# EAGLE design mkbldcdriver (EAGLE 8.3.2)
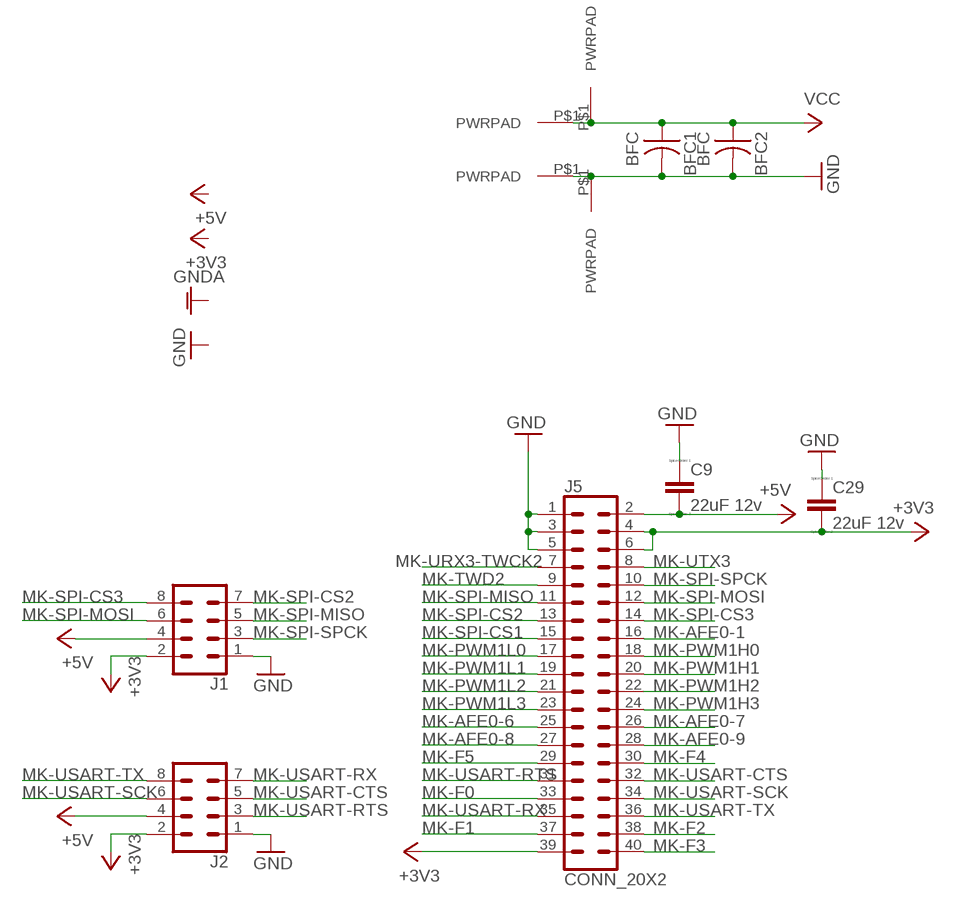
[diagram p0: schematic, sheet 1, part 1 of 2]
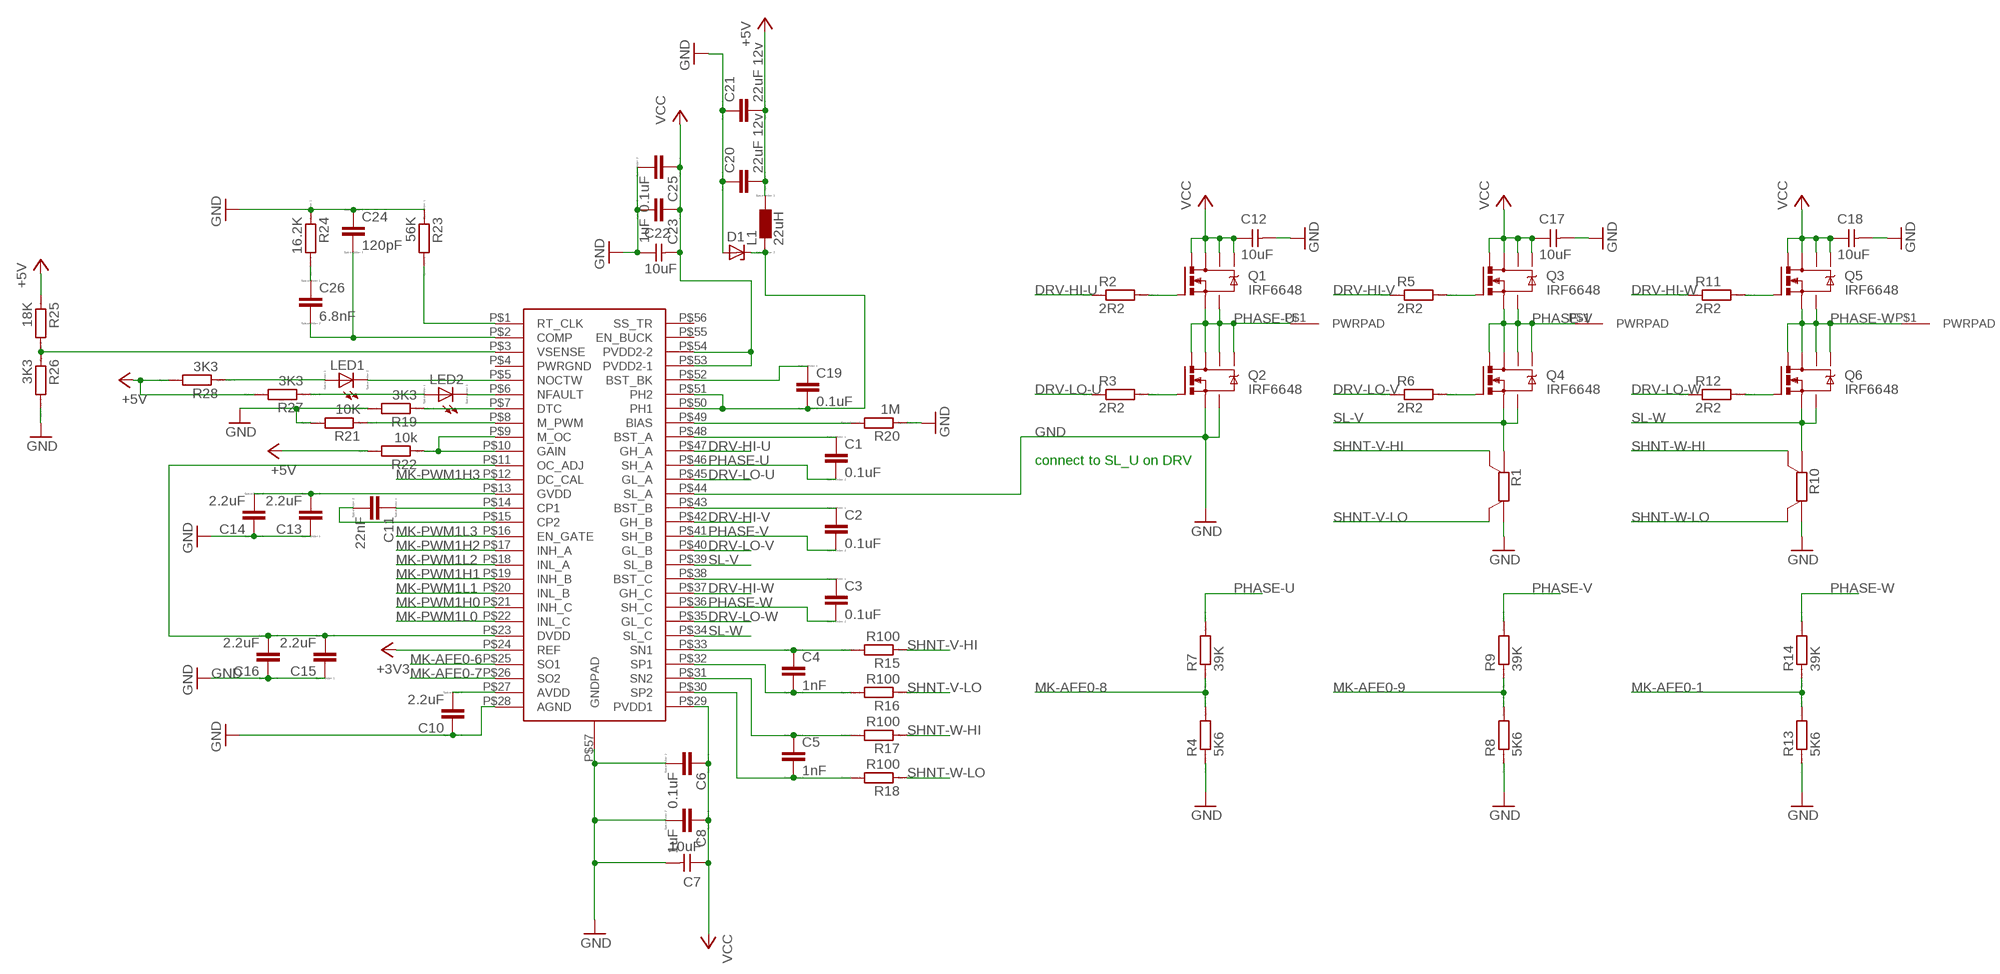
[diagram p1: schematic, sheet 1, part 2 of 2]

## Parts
BFC1  BFC  [BFC]
BFC2  BFC  [BFC]
C1  0.1uF  C  [C0805]
C2  0.1uF  C  [C0805]
C3  0.1uF  C  [C0805]
C4  1nF  C  [C0805]
C5  1nF  C  [C0805]
C6  0.1uF  C  [C0805]
C7  10uF  CAP-UNPOLARIZED2220  [C2220]
C8  1uF  C  [C0805]
C9  22uF 12v  C  [C0805]
C10  2.2uF  C  [C0805]
C11  22nF  C  [C0805]
C12  10uF  CAP-UNPOLARIZED2220  [C2220]
C13  2.2uF  C  [C0805]
C14  2.2uF  C  [C0805]
C15  2.2uF  C  [C0805]
C16  2.2uF  C  [C0805]
C17  10uF  CAP-UNPOLARIZED2220  [C2220]
C18  10uF  CAP-UNPOLARIZED2220  [C2220]
C19  0.1uF  C  [C0805]
C20  22uF 12v  C  [C0805]
C21  22uF 12v  C  [C0805]
C22  10uF  CAP-UNPOLARIZED2220  [C2220]
C23  1uF  C  [C0805]
C24  120pF  C  [C0805]
C25  0.1uF  C  [C0805]
C26  6.8nF  C  [C0805]
C29  22uF 12v  C  [C0805]
D1  ZENER_DIODESOD123  [SOD123]
J1  CONN_04X2SHROUDED  [2X4-SHROUDED]
J2  CONN_04X2SHROUDED  [2X4-SHROUDED]
J3  PWRPAD2-5MM  [PWRPAD_2-5MM]
J4  PWRPAD2-5MM  [PWRPAD_2-5MM]
J5  CONN_20X2  [2X20]
J6  PWRPAD2-5MM  [PWRPAD_2-5MM]
J7  PWRPAD4MM  [PWRPAD_4MM]
J8  PWRPAD4MM  [PWRPAD_4MM]
J9  PWRPAD4MM  [PWRPAD_4MM]
J10  PWRPAD4MM  [PWRPAD_4MM]
L1  22uH  L  [L1812]
LED1  LED_E  [LED_1206]
LED2  LED_E  [LED_1206]
Q1  IRF6648  [DIRECTFET]
Q2  IRF6648  [DIRECTFET]
Q3  IRF6648  [DIRECTFET]
Q4  IRF6648  [DIRECTFET]
Q5  IRF6648  [DIRECTFET]
Q6  IRF6648  [DIRECTFET]
R1  WSL2726  [WSL2726]
R2  2R2  R  [R0805]
R3  2R2  R  [R0805]
R4  5K6  R  [R0805]
R5  2R2  R  [R0805]
R6  2R2  R  [R0805]
R7  39K  R  [R0805]
R8  5K6  R  [R0805]
R9  39K  R  [R0805]
R10  WSL2726  [WSL2726]
R11  2R2  R  [R0805]
R12  2R2  R  [R0805]
R13  5K6  R  [R0805]
R14  39K  R  [R0805]
R15  R100  R  [R0805]
R16  R100  R  [R0805]
R17  R100  R  [R0805]
R18  R100  R  [R0805]
R19  3K3  R  [R0805]
R20  1M  R  [R0805]
R21  10K  R  [R0805]
R22  10k  R  [R0805]
R23  56K  R  [R0805]
R24  16.2K  R  [R0805]
R25  18K  R  [R0805]
R26  3K3  R  [R0805]
R27  3K3  R  [R0805]
R28  3K3  R  [R0805]
U$1  DRV8302  [HTSSOP-56]

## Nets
+3V3: C29.2 J1.2 J2.2 J5.4 J5.6 J5.39 U$1.P$24(REF)
+5V: C9.2 C20.2 C21.2 J1.4 J2.4 J5.2 L1.1 R22.2 R25.1 R27.2 R28.2
DRV-HI-U: R2.1 U$1.P$47(GH_A)
DRV-HI-V: R5.1 U$1.P$42(GH_B)
DRV-HI-W: R11.1 U$1.P$37(GH_C)
DRV-LO-U: R3.1 U$1.P$45(GL_A)
DRV-LO-V: R6.1 U$1.P$40(GL_B)
DRV-LO-W: R12.1 U$1.P$35(GL_C)
GND: BFC1.P$2 BFC2.P$2 C6.2 C7.2 C8.2 C9.1 C10.1 C12.2 C13.1 C14.1 C15.1 C16.1 C17.2 C18.2 C20.1 C21.1 C22.1 C23.2 C24.1 C25.2 C29.1 D1.ANODE J1.1 J2.1 J5.1 J5.3 J5.5 J8.P$1(PWRPAD) J10.P$1(PWRPAD) Q2.S@1(S) Q2.S@2(S) R1.A R4.1 R8.1 R10.A R13.1 R19.2 R20.1 R21.2 R23.1 R24.1 R26.2 U$1.P$28(AGND) U$1.P$44(SL_A) U$1.P$57(GNDPAD)
MK-AFE0-1: J5.16 R13.2 R14.1
MK-AFE0-6: J5.25 U$1.P$25(SO1)
MK-AFE0-7: J5.26 U$1.P$26(SO2)
MK-AFE0-8: J5.27 R4.2 R7.1
MK-AFE0-9: J5.28 R8.2 R9.1
MK-F0: J5.33
MK-F1: J5.37
MK-F2: J5.38
MK-F3: J5.40
MK-F4: J5.30
MK-F5: J5.29
MK-PWM1H0: J5.18 U$1.P$21(INH_C)
MK-PWM1H1: J5.20 U$1.P$19(INH_B)
MK-PWM1H2: J5.22 U$1.P$17(INH_A)
MK-PWM1H3: J5.24 U$1.P$12(DC_CAL)
MK-PWM1L0: J5.17 U$1.P$22(INL_C)
MK-PWM1L1: J5.19 U$1.P$20(INL_B)
MK-PWM1L2: J5.21 U$1.P$18(INL_A)
MK-PWM1L3: J5.23 U$1.P$16(EN_GATE)
MK-SPI-CS1: J5.15
MK-SPI-CS2: J1.7 J5.13
MK-SPI-CS3: J1.8 J5.14
MK-SPI-MISO: J1.5 J5.11
MK-SPI-MOSI: J1.6 J5.12
MK-SPI-SPCK: J1.3 J5.10
MK-TWD2: J5.9
MK-URX3-TWCK2: J5.7
MK-USART-CTS: J2.5 J5.32
MK-USART-RTS: J2.3 J5.31
MK-USART-RX: J2.7 J5.35
MK-USART-SCK: J2.6 J5.34
MK-USART-TX: J2.8 J5.36
MK-UTX3: J5.8
N$1: Q4.G R6.2
N$2: Q2.G R3.2
N$3: Q1.G R2.2
N$4: Q3.G R5.2
N$5: Q6.G R12.2
N$6: Q5.G R11.2
N$7: C3.1 U$1.P$38(BST_C)
N$8: C2.1 U$1.P$43(BST_B)
N$9: C1.1 U$1.P$48(BST_A)
N$11: C10.2 U$1.P$27(AVDD)
N$12: C11.1 U$1.P$14(CP1)
N$13: C4.1 R15.2 U$1.P$33(SN1)
N$14: C4.2 R16.2 U$1.P$32(SP1)
N$15: C5.1 R17.2 U$1.P$31(SN2)
N$16: C5.2 R18.2 U$1.P$30(SP2)
N$17: C11.2 U$1.P$15(CP2)
N$18: C13.2 C14.2 U$1.P$13(GVDD)
N$20: C15.2 C16.2 U$1.P$11(OC_ADJ) U$1.P$23(DVDD)
N$21: R19.1 U$1.P$7(DTC)
N$23: C19.1 U$1.P$52(BST_BK)
N$24: R20.2 U$1.P$49(BIAS)
N$25: R21.1 U$1.P$8(M_PWM)
N$26: R22.1 U$1.P$9(M_OC) U$1.P$10(GAIN)
N$27: C19.2 D1.CATHODE L1.2 U$1.P$50(PH1) U$1.P$51(PH2)
N$30: R23.2 U$1.P$1(RT_CLK)
N$31: C24.2 C26.2 U$1.P$2(COMP)
N$32: C26.1 R24.2
N$33: R25.2 R26.1 U$1.P$3(VSENSE)
N$35: LED1.C U$1.P$5(NOCTW)
N$36: LED2.C U$1.P$6(NFAULT)
N$37: LED2.A R27.1
N$38: LED1.A R28.1
PHASE-U: C1.2 J3.P$1(PWRPAD) Q1.S@1(S) Q1.S@2(S) Q2.D@1(D) Q2.D@2(D) Q2.D@3(D) Q2.D@4(D) R7.2 U$1.P$46(SH_A)
PHASE-V: C2.2 J4.P$1(PWRPAD) Q3.S@1(S) Q3.S@2(S) Q4.D@1(D) Q4.D@2(D) Q4.D@3(D) Q4.D@4(D) R9.2 U$1.P$41(SH_B)
PHASE-W: C3.2 J6.P$1(PWRPAD) Q5.S@1(S) Q5.S@2(S) Q6.D@1(D) Q6.D@2(D) Q6.D@3(D) Q6.D@4(D) R14.2 U$1.P$36(SH_C)
SHNT-V-HI: R1.SB R15.1
SHNT-V-LO: R1.SA R16.1
SHNT-W-HI: R10.SB R17.1
SHNT-W-LO: R10.SA R18.1
SL-V: Q4.S@1(S) Q4.S@2(S) R1.B U$1.P$39(SL_B)
SL-W: Q6.S@1(S) Q6.S@2(S) R10.B U$1.P$34(SL_C)
VCC: BFC1.P$1 BFC2.P$1 C6.1 C7.1 C8.1 C12.1 C17.1 C18.1 C22.2 C23.1 C25.1 J7.P$1(PWRPAD) J9.P$1(PWRPAD) Q1.D@1(D) Q1.D@2(D) Q1.D@3(D) Q1.D@4(D) Q3.D@1(D) Q3.D@2(D) Q3.D@3(D) Q3.D@4(D) Q5.D@1(D) Q5.D@2(D) Q5.D@3(D) Q5.D@4(D) U$1.P$29(PVDD1) U$1.P$53(PVDD2-1) U$1.P$54(PVDD2-2)
Unconnected: U$1.P$4(PWRGND) U$1.P$55(EN_BUCK) U$1.P$56(SS_TR)

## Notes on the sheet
- connect to SL_U on DRV

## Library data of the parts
BFC1 BFC2 = fab:BFC
C1-C6 C8-C11 C13-C16 C19-C21 C23-C26 C29 = eagle-ltspice:C: CAPACITOR, European symbol; SPICEMODEL: NONE; SPICEPREFIX: C
C7 C12 C17 C18 C22 = fab:CAP-UNPOLARIZED
D1 = fab:ZENER_DIODE: zener diode
J1 J2 = fab:CONN_04X2: Multi connection point. Often used as Generic Header-pin footprint for 0.1 inch spaced/style header connections On any of the 0.1 inch spaced packages, you can populate with these: Break Away Headers - Straight (PRT-00116) Break Away Male Headers - Right Angle (PRT-00553) Female Headers (PRT-00115)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
J3 J4 J6-J10 = fab:PWRPAD
J5 = SparkFun-Connectors:CONN_20X2: Multi connection point. Often used as Generic Header-pin footprint for 0.1 inch spaced/style header connections On any of the 0.1 inch spaced packages, you can populate with these: Break Away Headers - Straight (PRT-00116) Break Away Male Headers - Right Angle (PRT-00553) Female Headers (PRT-00115)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
L1 = eagle-ltspice:L: INDUCTOR, European symbol; SPICEMODEL: NONE; SPICEPREFIX: L
LED1 LED2 = eagle-ltspice:LED_E: LED; SPICEMODEL: NONE; SPICEPREFIX: D; SPICETYPE: diode
Q1-Q6 = transistor-power:IRF6648: DirectFET Power MOSFET Source: http://www.irf.com/product-info/datasheets/data/irf6648.pdf
R1 R10 = fab:WSL2726: SMD SHUNT RESISTOR
R2-R9 R11-R28 = eagle-ltspice:R: RESISTOR, European symbol; SPICEMODEL: NONE; SPICEPREFIX: R
U$1 = fab:DRV8302

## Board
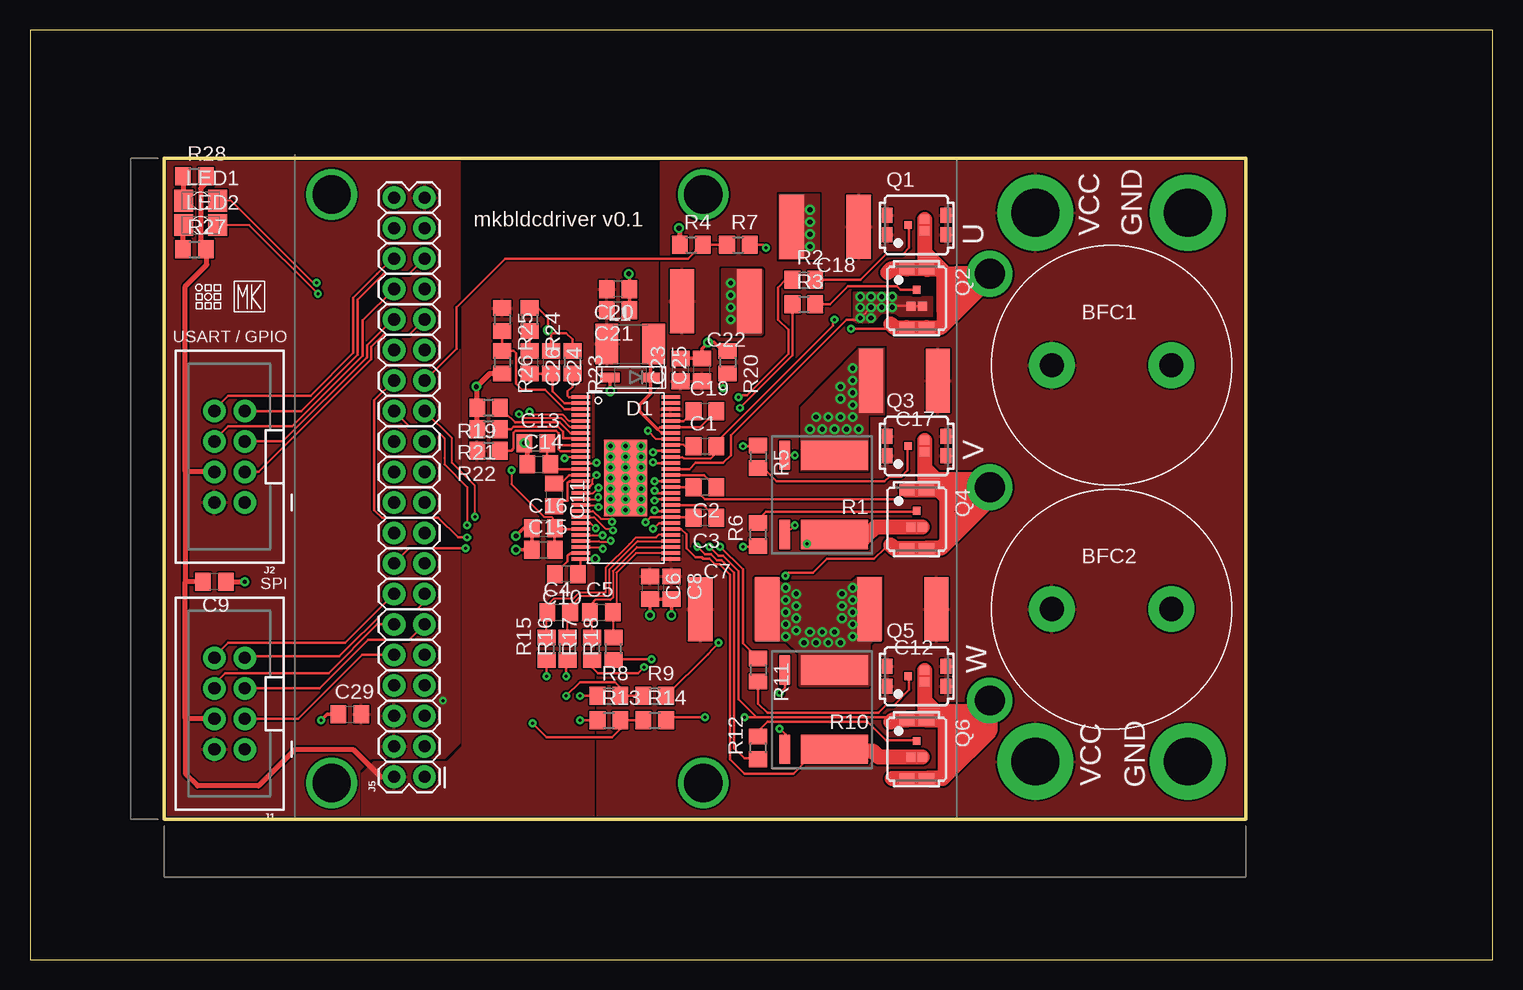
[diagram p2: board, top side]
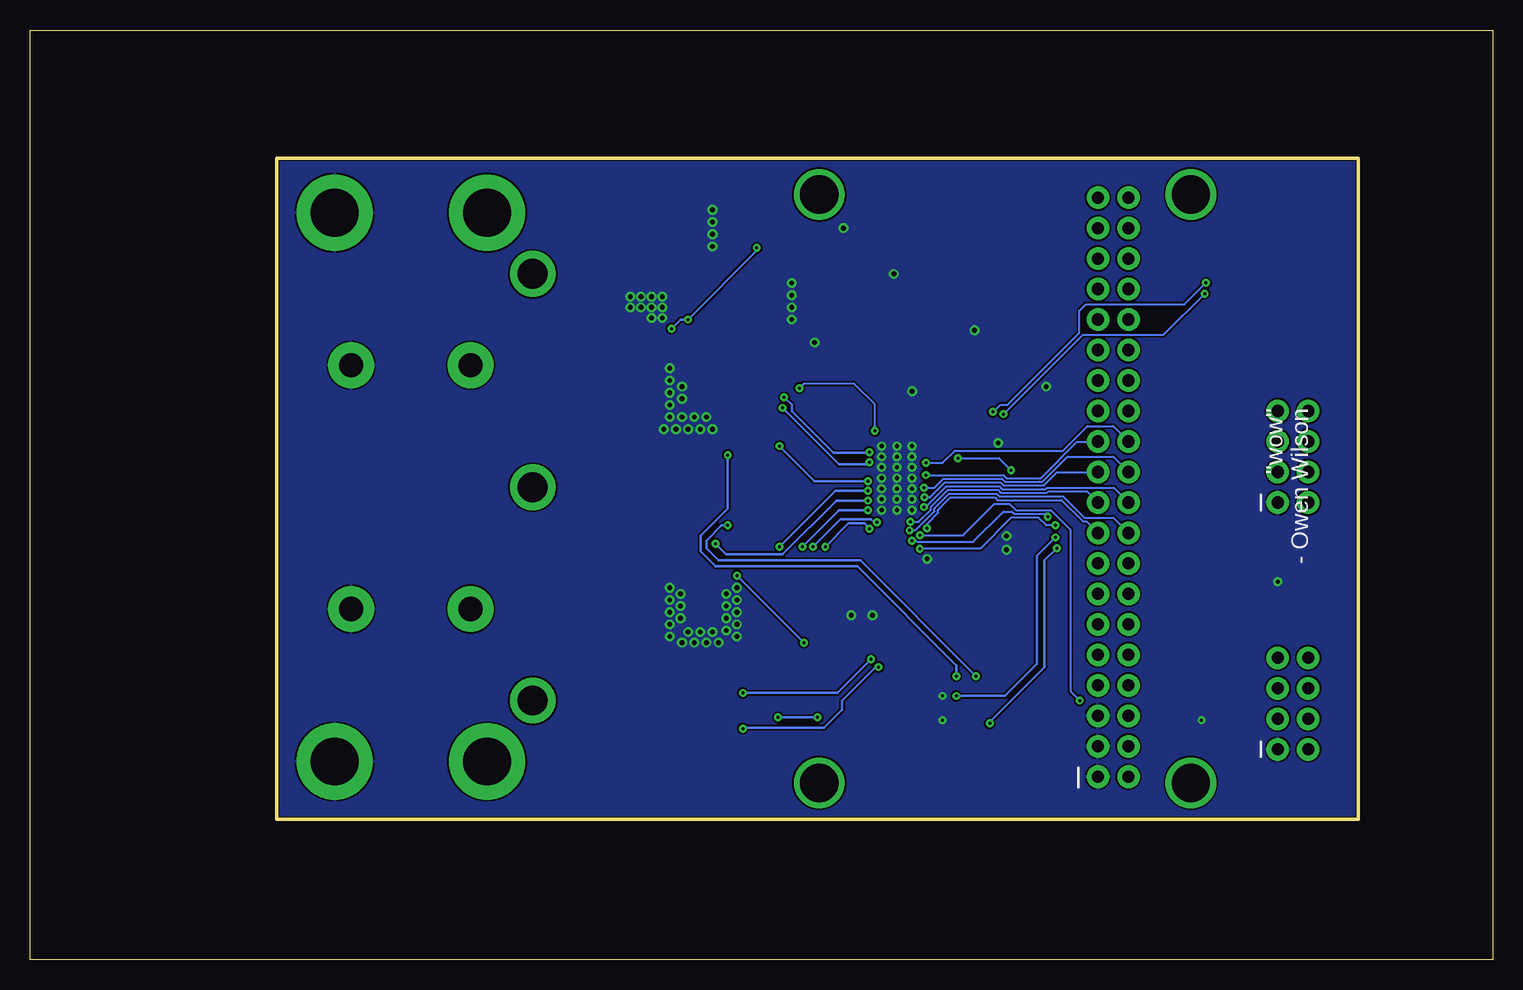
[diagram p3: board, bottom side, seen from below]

Size 121.92 x 77.47 mm. Coordinates in mm from the lower left corner, seen from the top.
Outline: 0,0 121.92,0 121.92,77.47 0,77.47 0,0
Outline: 11.18,66.8 11.18,11.68 101.35,11.68 101.35,66.8 11.18,66.8
Copper layers (1*16): Top 0.035mm / dielectric 1.5mm / Bottom 0.035mm
Design rules "default *": minimum track width 6mil, minimum drill 0.35mm, track to track 6mil, track to pad 6mil, pad to pad 6mil, via to via 6mil, smd to smd 6mil, copper to edge 6mil, drill to drill 6mil, minimum pad ring 10mil, minimum via ring 8mil, stop-mask expansion 4mil, vias tented up to drill 0mil, thermal gap 6mil
Milling: 4 lines

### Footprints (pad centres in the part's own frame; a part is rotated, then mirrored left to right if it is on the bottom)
BFC = drill 2.032 pad 3.81: P$1 -4.978,0; P$2 4.978,0
C0805 = smd 1.3 x 1.5: 1 -0.95,0; 2 0.95,0
C2220 = smd 2.032 x 5.334: 1 -2.794,0; 2 2.794,0
SOD123 = smd 1.6 x 0.8: ANODE 1.7,0; CATHODE -1.7,0
2X4-SHROUDED = drill 1.016 pad 1.88: 1 -1.27,2.54; 2 1.27,2.54; 3 -1.27,0; 4 1.27,0; 5 -1.27,-2.54; 6 1.27,-2.54; 7 -1.27,-5.08; 8 1.27,-5.08
PWRPAD_2-5MM = drill 2.489 pad 3.81: P$1 0,0
2X20 = drill 1.016 pad 1.88: 1 0,0; 2 0,2.54; 3 2.54,0; 4 2.54,2.54; 5 5.08,0; 6 5.08,2.54; 7 7.62,0; 8 7.62,2.54; 9 10.16,0; 10 10.16,2.54; 11 12.7,0; 12 12.7,2.54; 13 15.24,0; 14 15.24,2.54; 15 17.78,0; 16 17.78,2.54; 17 20.32,0; 18 20.32,2.54; 19 22.86,0; 20 22.86,2.54; 21 25.4,0; 22 25.4,2.54; 23 27.94,0; 24 27.94,2.54; 25 30.48,0; 26 30.48,2.54; 27 33.02,0; 28 33.02,2.54; 29 35.56,0; 30 35.56,2.54; 31 38.1,0; 32 38.1,2.54; 33 40.64,0; 34 40.64,2.54; 35 43.18,0; 36 43.18,2.54; 37 45.72,0; 38 45.72,2.54; 39 48.26,0; 40 48.26,2.54
PWRPAD_4MM = drill 3.988 pad 6.35: P$1 0,0
L1812 = smd 1.9 x 3.4: 1 -1.95,0; 2 1.95,0
LED_1206 = smd 1.6 x 1.803: A -1.422,0; C 1.422,0
DIRECTFET = smd 0.9 x 1.25: D@1 -2.45,0.825; D@2 -2.45,-0.825; D@3 2.45,0.825; D@4 2.45,-0.825 | smd 0.65 x 0.65: G -0.7,0 | smd 0.75 x 0.75: S@1 0.65,0.475; S@2 0.65,-0.475
WSL2726 = smd 2.438 x 5.588: A 3.302,2.794; B -3.302,2.794 | smd 2.438 x 0.889: SA 3.302,6.921; SB -3.302,6.921
R0805 = smd 1.3 x 1.5: 1 -0.95,0; 2 0.95,0
HTSSOP-56 = smd 1.549 x 0.279: P$1 -3.75,6.75; P$2 -3.75,6.25; P$3 -3.75,5.75; P$4 -3.75,5.25; P$5 -3.75,4.75; P$6 -3.75,4.25; P$7 -3.75,3.75; P$8 -3.75,3.25; P$9 -3.75,2.75; P$10 -3.75,2.25; P$11 -3.75,1.75; P$12 -3.75,1.25; P$13 -3.75,0.75; P$14 -3.75,0.25; P$15 -3.75,-0.25; P$16 -3.75,-0.75; P$17 -3.75,-1.25; P$18 -3.75,-1.75; P$19 -3.75,-2.25; P$20 -3.75,-2.75; P$21 -3.75,-3.25; P$22 -3.75,-3.75; P$23 -3.75,-4.25; P$24 -3.75,-4.75; P$25 -3.75,-5.25; P$26 -3.75,-5.75; P$27 -3.75,-6.25; P$28 -3.75,-6.75; P$29 3.75,-6.75; P$30 3.75,-6.25; P$31 3.75,-5.75; P$32 3.75,-5.25; P$33 3.75,-4.75; P$34 3.75,-4.25; P$35 3.75,-3.75; P$36 3.75,-3.25; P$37 3.75,-2.75; P$38 3.75,-2.25; P$39 3.75,-1.75; P$40 3.75,-1.25; P$41 3.75,-0.75; P$42 3.75,-0.25; P$43 3.75,0.25; P$44 3.75,0.75; P$45 3.75,1.25; P$46 3.75,1.75; P$47 3.75,2.25; P$48 3.75,2.75; P$49 3.75,3.25; P$50 3.75,3.75; P$51 3.75,4.25; P$52 3.75,4.75; P$53 3.75,5.25; P$54 3.75,5.75; P$55 3.75,6.25; P$56 3.75,6.75 | smd 3.581 x 6.35: P$57 0,0

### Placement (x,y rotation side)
BFC1  90.17,49.53 0 top
BFC2  90.17,29.21 0 top
C1  56.26,42.8 0 top
C2  56.26,39.37 180 top
C3  56.26,36.83 180 top
C4  44.07,28.96 0 top
C5  47.62,28.96 0 top
C6  51.69,30.99 270 top
C7  58.67,29.21 0 top
C8  53.47,30.99 270 top
C9  15.37,31.5 180 top
C10  44.7,32.13 180 top
C11  43.69,38.73 270 top
C12  72.77,29.21 180 top
C13  42.16,43.05 0 top
C14  42.42,41.27 0 top
C15  42.8,34.16 0 top
C16  42.8,35.94 0 top
C17  72.9,48.26 180 top
C18  66.29,61.09 180 top
C19  56.26,45.72 0 top
C20  49.02,55.88 180 top
C21  49.02,54.1 180 top
C22  57.15,54.86 180 top
C23  54.23,49.15 90 top
C24  43.43,49.78 270 top
C25  56.01,49.15 90 top
C26  41.66,49.78 270 top
C29  26.67,20.45 0 top
D1  50.04,48.51 180 top
J1  16.64,20.07 180 top
J2  16.64,40.64 180 top
J3  80.01,57.15 0 top
J4  80.01,39.37 0 top
J5  32.89,15.24 90 top
J6  80.01,21.59 0 top
J7  83.82,62.23 0 top
J8  96.52,62.23 0 top
J9  83.82,16.51 0 top
J10  96.52,16.51 0 top
L1  50.04,51.31 0 top
LED1  14.22,63.25 0 top
LED2  14.22,61.21 0 top
Q1  73.91,61.21 0 top
Q2  73.91,55.12 270 top
Q3  73.91,42.8 0 top
Q4  73.91,36.7 270 top
Q5  73.91,23.62 0 top
Q6  73.91,17.53 270 top
R1  69.85,38.73 90 top
R2  64.52,56.64 0 top
R3  64.52,54.61 0 top
R4  55.12,59.56 0 top
R5  60.71,41.91 270 top
R6  60.71,35.43 90 top
R7  59.05,59.56 0 top
R8  48.26,21.97 0 top
R9  52.07,21.97 0 top
R10  69.85,20.83 90 top
R11  60.71,24.13 270 top
R12  60.71,17.65 90 top
R13  48.26,19.94 0 top
R14  52.07,19.94 0 top
R15  43.05,25.91 90 top
R16  44.83,25.91 90 top
R17  46.86,25.91 90 top
R18  48.64,25.91 90 top
R19  38.23,45.97 180 top
R20  58.17,49.78 270 top
R21  38.23,44.2 180 top
R22  38.23,42.42 180 top
R23  45.21,49.78 270 top
R24  41.66,53.34 270 top
R25  39.37,53.34 270 top
R26  39.37,49.78 270 top
R27  13.72,59.18 0 top
R28  13.72,65.28 0 top
U$1  49.66,40.13 0 top
U$2  [CBA-SILK-LOGO]  14.86,55.24 0 top
U$3  [MK-LOGO-SILK]  18.29,55.24 0 top

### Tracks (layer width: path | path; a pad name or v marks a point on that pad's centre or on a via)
+3V3  (via drill 0.25)
  Top 0.152: U$1.P$24 46.93,35.38 47.72,35.38 v47.73,35.36
  Bottom 0.152: v47.73,35.36 44.14,35.36 41.66,37.85 41.53,37.97 40.26,37.97 39.75,37.47 36.83,37.47 35.18,35.81 35.18,22.35 v34.42,21.59
  pour Top: 35.81,66.8 35.81,18.03 34.54,16.76 28.45,16.76 27.43,15.75 27.43,11.68 11.18,11.68 11.18,66.8
+5V
  Top 0.406: J5.2 29.21,15.24 26.92,17.53 22.1,17.53 19.05,14.48 13.97,14.48 12.95,15.49 12.95,20.07 | 12.95,20.07 12.95,31.5 | C9.2 12.95,31.5 | J1.4 12.95,20.07 | 12.95,40.64 12.95,31.5 | 12.95,40.64 12.95,56.13 14.73,57.91 14.73,59.12 R27.2 14.22,59.62 14.22,64.26 14.67,64.7 R28.2 | J2.4 12.95,40.64
  pour Top: 52.32,66.8 52.32,48.01 51.56,47.24 46.99,47.24 46.99,11.94 46.99,11.68 27.69,11.68 27.69,15.49 28.7,16.51 34.8,16.51 36.07,17.78 36.07,66.8
DRV-HI-U  (via drill 0.25)
  Top 0.203: v59.05,46.86 59.24,47.05 59.76,47.05 63.21,50.51 63.21,52.49 62.36,53.34 62.36,56.01 62.99,56.64 R2.1 | v51.94,42.29 52.07,42.29 52.2,42.42 53.37,42.42 U$1.P$47
  Bottom 0.203: v59.05,46.86 58.42,46.23 58.42,45.72 54.93,42.23 52.01,42.23 v51.94,42.29
DRV-HI-V  (via drill 0.25)
  Top 0.203: U$1.P$42 v52.07,39.88 | v59.44,42.8 60.65,42.8 R5.1
  Bottom 0.203: v52.07,39.88 56.52,39.88 v59.44,42.8
DRV-HI-W  (via drill 0.25)
  Top 0.203: U$1.P$37 52.14,37.38 v52.07,37.45 | R11.1 59.44,26.35 59.44,32.51 v57.53,34.42
  Bottom 0.203: v52.07,37.45 54.5,37.45 v57.53,34.42
DRV-LO-U  (via drill 0.25)
  Top 0.203: U$1.P$45 52.02,41.38 v51.94,41.46 | R3.1 63.57,50.36 v59.18,45.97
  Bottom 0.203: v59.18,45.97 54.48,41.27 52.13,41.27 v51.94,41.46
DRV-LO-V  (via drill 0.25)
  Top 0.203: U$1.P$40 52.26,38.88 v52.07,39.07 | v59.44,34.42 60.64,34.42 R6.1
  Bottom 0.203: v52.07,39.07 54.78,39.07 v59.44,34.42
DRV-LO-W  (via drill 0.25)
  Top 0.203: R12.1 60.65,16.76 59.56,16.76 58.7,17.63 58.7,32.23 57.85,33.08 57.85,33.09 57.64,33.3 57.26,33.3 56.77,33.78 56.26,33.78 v55.63,34.42 | U$1.P$35 52.43,36.38 v51.94,35.89
  Bottom 0.203: v51.94,35.89 51.94,35.94 52.35,36.35 53.7,36.35 v55.63,34.42
GND  (via drill 0.25, 0.35, 0.4)
  Top 0.152: U$1.P$28 47.11,33.38 v47.12,33.4
  Top 0.203: R24.1 42.36,54.29 43.18,53.47 v43.18,52.45 43.43,52.2 | C24.1 43.43,52.2 | R23.1 45.21,51.69 44.7,52.2 43.43,52.2 | U$1.P$28 45.91,32.13 C10.1 | 51.07,40.88 v50.93,41.02 | U$1.P$44 54.98,40.88 55.5,41.4 57.78,41.4 58.42,42.04 58.42,43.69 68.07,53.34 69.09,53.34 70.23,54.48 73.42,54.48 Q2.S@2 Q2.S@1 | R13.1 v45.85,19.94 | R8.1 v45.85,21.97
  Top 0.305: D1.ANODE 48.34,47.42 v48.39,47.37 | C21.1 C20.1 49.97,57.09 v49.91,57.15 | C23.2 C25.2 56.01,50.93 v56.52,51.44 57.02,51.44 57.72,50.73 R20.1 | v51.69,28.7 C6.2 C8.2 v53.47,28.7 | v40.51,34.16 C15.1 C16.1 41.15,35.94 v40.51,35.31 | C29.1 24.77,20.45 v24.26,19.94
  Top 0.406: C9.1 v17.91,31.5 | C14.1 41.47,42.8 C13.1 | R21.2 R19.2 37.28,47.69 v37.21,47.75 38.29,48.83 R26.2 | R4.1 54.17,60.89 v54.1,60.96
  other vias: 48.39,42.8 49.66,42.8 50.93,42.8 48.39,41.91 48.39,41.02 48.39,40.13 48.39,38.35 48.39,39.24 48.39,37.47 49.66,41.91 49.66,41.02 50.93,41.91 50.93,40.13 49.66,40.13 49.66,39.24 49.66,38.35 49.66,37.47 50.93,39.24 50.93,38.35 50.93,37.47 41.21,43.05 63.88,30.48 62.99,29.97 62.99,28.96 62.99,27.94 62.99,26.92 68.58,26.92 68.58,27.94 68.58,28.96 68.58,29.97 68.58,30.99 67.56,26.42 66.55,26.42 65.53,26.42 64.52,26.42 65.02,27.3 69.09,44.2 68.07,44.2 67.06,44.2 66.04,44.2 65.02,44.2 68.58,49.28 68.58,48.26 68.58,47.24 68.58,46.23 67.56,46.74 67.56,45.21 65.02,59.44 65.02,60.45 65.02,61.47 65.02,62.48 58.42,56.39 58.42,55.37 58.42,54.36 58.42,53.34 66.55,45.21 65.53,45.21 68.58,45.21 67.56,47.75 71.88,55.24 71.88,54.36 70.99,54.36 70.99,55.24 70.1,55.24 70.1,54.36 70.1,53.47 69.22,53.47 69.22,54.36 69.22,55.24 63.88,27.43 63.88,28.45 63.88,29.46 66.04,27.3 67.06,27.3 67.69,28.45 67.69,29.46 67.69,30.48 62.99,30.99
  pour Bottom: 11.18,66.8 101.35,66.8 101.35,11.68 11.18,11.68
  pour Top (isolate 0.254, no thermals): 64.14,22.86 64.14,25.53 63.12,26.54 60.58,26.54 60.45,26.67 60.45,31.75 60.58,31.88 62.23,31.88 62.61,31.5 68.58,31.5 68.96,31.88 70.99,31.88 70.99,26.67 70.87,26.54 70.23,26.54 69.98,26.29 69.98,22.86 69.85,22.73 64.26,22.73
  pour Top (isolate 0.254, no thermals): 62.48,63.75 62.48,58.42 65.79,58.42 65.79,63.75
  pour Top (isolate 0.254, no thermals): 60.96,57.53 57.66,57.53 57.66,52.07 60.96,52.07 61.09,52.2 61.09,57.4
  pour Top (isolate 0.254, no thermals): 71.25,50.93 69.09,50.93 64.26,45.97 64.26,40.77 69.85,40.77 69.85,45.47 71.25,45.47
  pour Top (isolate 0.254, no thermals): 72.39,55.24 75.31,55.24 75.31,53.59 72.39,53.59 72.14,53.85 70.99,53.85 70.23,53.09 68.71,53.09 68.71,55.63 72.01,55.63
MK-AFE0-1  (via drill 0.25)
  Top 0.203: R14.1 R13.2 49.21,19.24 48.51,18.54 43.05,18.54 v41.91,19.68 | v36.32,34.29 31.62,34.29 J5.16
  Bottom 0.203: v41.91,19.68 41.91,19.81 37.34,24.38 37.34,33.27 v36.32,34.29
MK-AFE0-6  (via drill 0.25)
  Top 0.152: U$1.P$25 47.43,34.88 47.5,34.81 48.32,34.81 v48.41,34.9 | J5.25 35.18,43.43 35.18,41.4 37.08,39.5 v37.08,36.91
  Bottom 0.152: v48.41,34.9 48.06,34.9 47.97,34.81 43.3,34.81 40.77,37.34 40.05,37.34 39.88,37.16 37.34,37.16 v37.08,36.91
MK-AFE0-7  (via drill 0.25)
  Top 0.152: U$1.P$26 47.62,34.38 v47.75,34.25 | J5.26 31.62,44.45 33.53,44.45 34.54,43.43 34.54,41.78 34.54,41.27 36.45,39.37 v36.45,36.2
  Bottom 0.152: v47.75,34.25 42.71,34.25 40.13,36.83 37.85,36.83 37.21,36.2 v36.45,36.2
MK-AFE0-8
  Top 0.203: R7.1 R4.2 56.01,59.56 54.86,58.42 39.62,58.42 35.56,54.36 35.56,50.93 J5.27
MK-AFE0-9  (via drill 0.25)
  Top 0.203: R9.1 R8.2 49.21,22.67 48.77,23.11 45.85,23.11 v44.7,21.97 | v36.45,35.18 35.69,35.18 34.04,36.83 29.34,36.83 28.7,37.47 28.7,46.61 J5.28
  Bottom 0.203: v44.7,21.97 40.64,21.97 37.97,24.64 37.97,33.66 v36.45,35.18
MK-PWM1H0  (via drill 0.25)
  Top 0.152: v48.59,35.76 48.44,35.92 47.97,35.92 47,36.88 U$1.P$21
  Bottom 0.152: J5.18 31.62,36.83 34.04,36.83 35.81,38.61 41.14,38.61 41.36,38.83 45.3,38.83 46.52,37.6 46.52,37.36 48.12,35.76 v48.59,35.76
MK-PWM1H1  (via drill 0.25)
  Top 0.152: U$1.P$19 47.22,37.88 v47.39,37.72
  Bottom 0.152: v47.39,37.72 47.27,37.72 45.54,39.45 41.12,39.45 40.89,39.22 37.52,39.22 | 37.52,39.22 | 37.52,39.22 37.26,39.22 37.16,39.32 31.57,39.32 J5.20
MK-PWM1H2  (via drill 0.25)
  Top 0.152: U$1.P$17 46.93,38.88 v47.39,39.34
  Bottom 0.152: v47.39,39.34 46.52,39.34 45.77,40.08 40.89,40.08 40.64,39.83 37.8,39.83 | 37.8,39.83 | 37.8,39.83 37.52,39.83 35.43,41.91 31.62,41.91 J5.22
MK-PWM1H3  (via drill 0.25)
  Top 0.152: U$1.P$12 47.22,41.38 v47.24,41.4
  Bottom 0.152: v47.24,41.4 45.85,41.4 44.83,42.42 35.81,42.42 33.78,44.45 31.62,44.45 J5.24
MK-PWM1L0  (via drill 0.25)
  Top 0.152: U$1.P$22 46.72,36.38 v47.16,35.94
  Bottom 0.152: v47.16,35.94 47.16,36.29 46.22,37.23 46.22,37.47 46.1,37.59 46.1,37.6 45.18,38.52 41.49,38.52 41.27,38.3 35.94,38.3 34.16,36.52 33.86,36.52 J5.17
MK-PWM1L1  (via drill 0.25)
  Top 0.152: U$1.P$20 46.93,37.38 47.59,36.73 48.26,36.73 v48.51,36.48
  Bottom 0.152: J5.19 33.81,39.02 37.03,39.02 37.14,38.91 41.02,38.91 41.25,39.14 45.42,39.14 46.83,37.73 46.83,37.49 47.84,36.48 v48.51,36.48
MK-PWM1L2  (via drill 0.25)
  Top 0.152: U$1.P$18 47.23,38.38 v47.37,38.53
  Bottom 0.152: v47.37,38.53 46.89,38.53 45.65,39.78 41.02,39.78 40.77,39.52 37.92,39.52 | 37.92,39.52 | 37.92,39.52 37.39,39.52 36.3,40.62 32.92,40.62 J5.21
MK-PWM1L3  (via drill 0.25)
  Top 0.152: v47.24,40.39 46.91,40.05 46.91,39.65 46.65,39.38 U$1.P$16
  Bottom 0.152: v47.24,40.39 40.77,40.39 40.51,40.13 37.67,40.13 34.65,43.16 32.92,43.16 J5.23
MK-SPI-CS2
  Top 0.203: J5.13 32.89,29.84 32.26,29.21 29.72,29.21 25.78,25.27 18.03,25.27 J1.7
MK-SPI-CS3
  Top 0.203: J1.8 15.37,25.27 16.51,26.42 26.29,26.42 J5.14
MK-SPI-MISO
  Top 0.203: J1.5 24.13,22.61 28.19,26.67 31.62,26.67 J5.11
MK-SPI-MOSI
  Top 0.203: J1.6 15.37,22.99 16.26,23.88 24.89,23.88 28.96,27.94 J5.12
MK-SPI-SPCK
  Top 0.203: J1.3 22.35,20.07 27.69,25.4 J5.10
MK-USART-CTS
  Top 0.203: J5.32 30.23,53.34 28.09,51.2 28.09,50.19 28.07,50.16 28.06,50.16 21.08,43.18 J2.5
MK-USART-RTS
  Top 0.203: J2.3 19.05,40.64 28.45,50.04 28.45,51.05 29.46,52.07 31.62,52.07 J5.31
MK-USART-RX
  Top 0.203: J2.7 22.62,45.72 27.31,50.41 27.31,52.32 | 27.31,52.32 27.31,52.46 | J5.35 31.62,57.15 29.46,57.15 27.31,55 27.31,52.32
MK-USART-SCK
  Top 0.203: J2.6 15.37,43.31 16.51,44.45 21.85,44.45 27.74,50.34 27.74,53.26 J5.34
MK-USART-TX
  Top 0.203: J5.36 30.23,58.42 28.96,57.15 26.95,55.14 26.95,50.56 23.38,46.99 16.51,46.99 15.37,45.85 J2.8
N$1
  Top 0.203: R6.2 60.71,36.7 61.34,37.34 73.85,37.34 Q4.G
N$2
  Top 0.203: Q2.G 72.58,55.82 72.26,56.13 68.2,56.13 66.67,54.61 R3.2
N$3
  Top 0.203: Q1.G 73.28,61.15 73.28,59.31 72.77,58.8 71.37,58.8 69.22,56.64 R2.2
N$4
  Top 0.203: R5.2 61.15,40.96 62.23,39.88 71.25,39.88 71.63,40.26 72.64,40.26 73.15,40.77 73.15,42.74 Q3.G
N$5
  Top 0.203: R12.2 60.71,19.05 61.49,19.84 69.83,19.84 71.37,18.29 73.85,18.29 Q6.G
N$6
  Top 0.203: Q5.G 73.28,23.56 73.28,22.48 72.01,21.21 71.37,21.21 70.74,20.57 61.47,20.57 60.71,21.34 R11.2
N$7
  Top 0.203: U$1.P$38 56.16,37.88 C3.1
N$8
  Top 0.203: U$1.P$43 56.2,40.38 C2.1
N$9
  Top 0.152: C1.1 54.61,42.8 54.48,42.93 53.45,42.93 U$1.P$48
N$11
  Top 0.203: U$1.P$27 45.06,33.88 44.83,33.66 44.83,33.21 C10.2
N$12
  Top 0.203: C11.1 44.26,39.69 44.96,40.39 U$1.P$14
N$13
  Top 0.152: 49.98,34.63 | 49.98,34.63 47.98,32.64 47.98,30.58 45.77,30.58 45.25,30.06 43.65,30.06 43.05,29.46 43.05,29.02 C4.1 43.05,28.89 R15.2 | 49.98,34.63 | 49.98,34.63 50.53,35.19 52.2,35.19 52.45,35.43 53.36,35.43 U$1.P$33
N$14
  Top 0.152: 50.28,34.51 | 50.28,34.51 50.66,34.88 U$1.P$32 | 50.28,34.51 48.28,32.51 48.28,30.38 48.18,30.28 45.9,30.28 45.09,29.46 45.09,29.02 C4.2 44.83,28.77 R16.2
N$15
  Top 0.152: R17.2 46.86,28.77 C5.1 46.86,29.14 46.86,29.72 47.12,29.97 48.39,29.97 48.59,30.18 48.59,32.38 50.59,34.38 U$1.P$31
N$16
  Top 0.152: U$1.P$30 50.52,33.88 48.9,32.26 48.9,29.28 C5.2 48.64,28.89 R18.2
N$17
  Top 0.203: U$1.P$15 44.96,39.88 44.83,39.75 44.83,38.23 44.13,38.23 C11.2
N$18
  Top 0.203: C13.2 43.11,41.91 C14.2 43.76,40.88 U$1.P$13
N$20  (via drill 0.25)
  Top 0.152: U$1.P$11 44.68,41.88 v44.58,41.78 | v40.13,40.77 40.13,39.62 42.84,36.91 43.48,36.91 43.56,36.83 43.56,36.13 C16.2
  Top 0.203: U$1.P$23 43.81,35.88 C16.2 C15.2
  Bottom 0.152: v44.58,41.78 41.15,41.78 v40.13,40.77
N$21
  Top 0.203: U$1.P$7 45.05,43.88 44.16,44.77 40.45,44.77 39.62,45.59 39.62,45.78 R19.1
N$23
  Top 0.203: U$1.P$52 54.47,44.88 C19.1
N$24  (via drill 0.25)
  Top 0.152: U$1.P$49 52.19,43.38 v51.5,44.07 | v57.78,47.62 57.78,48.45 R20.2
  Bottom 0.152: v51.5,44.07 51.5,46.29 53.21,48.01 57.4,48.01 v57.78,47.62
N$25
  Top 0.203: R21.1 40.09,44.2 40.31,44.41 43.56,44.41 44.02,44.41 44.42,44.01 44.42,43.43 45.85,43.43 U$1.P$8
N$26
  Top 0.203: U$1.P$10 44.23,42.38 44.07,42.55 44.07,42.8 | 44.07,42.8 44.07,43.86 43.87,44.06 40.46,44.06 40.31,43.91 40.31,42.6 40.13,42.42 R22.1 | U$1.P$9 44.15,42.88 44.07,42.8
N$27
  Top 0.152: C19.2 57.4,45.72 | 53.47,44.32 U$1.P$51
  Top 0.203: U$1.P$50 52.64,43.88 52.32,44.2 52.51,44.38 U$1.P$51 55.87,44.38 C19.2
  Top 0.305: L1.2 51.74,51.06 D1.CATHODE 51.74,47.17 50.8,46.23 50.8,45.72 52.32,44.2
N$30
  Top 0.203: R23.2 45.21,47.75 44.83,47.37 44.83,46.99 44.96,46.86 45.89,46.86 U$1.P$1
N$31
  Top 0.203: C26.2 C24.2 43.56,48.71 43.56,47.37 44.55,46.38 U$1.P$2
N$32
  Top 0.203: C26.1 R24.2
N$33
  Top 0.203: R25.2 R26.1 40.33,50.73 40.51,50.55 40.51,48.01 41.02,47.5 42.93,47.5 44.58,45.85 45.87,45.85 U$1.P$3
N$35  (via drill 0.25)
  Top 0.152: U$1.P$5 44.95,44.88 44.43,45.4 41.91,45.4 v41.66,45.66 | LED1.C 16.76,63.25 23.61,56.4 v23.89,56.4
  Bottom 0.152: v41.66,45.66 41.59,45.66 41.02,46.23 40.44,46.23 34.44,52.22 34.44,54.08 33.91,54.61 25.68,54.61 v23.89,56.4
N$36  (via drill 0.25)
  Top 0.152: U$1.P$6 45.02,44.38 44.3,45.1 41.13,45.1 v40.77,45.47 | v24,55.5 18.29,61.21 LED2.C
  Bottom 0.152: v24,55.5 27.43,52.07 34.16,52.07 v40.77,45.47
N$37
  Top 0.406: R27.1 12.77,61.18 LED2.A
N$38
  Top 0.406: LED1.A 12.8,65.24 R28.1
N$41  (via drill 3.2)
  other vias: 56.13,14.73
N$42  (via drill 3.2)
  other vias: 56.13,63.75
N$43  (via drill 3.2)
  other vias: 25.15,14.73
N$44  (via drill 3.2)
  other vias: 25.15,63.75
PHASE-U  (via drill 0.25)
  Top 0.152: U$1.P$46 54.38,41.88 54.48,41.78 56.77,41.78 57.02,42.04 57.02,42.61 C1.2
  Top 0.203: C1.2 57.21,43.11 66.93,52.83 66.93,53.21 v67.06,53.34 | 71.88,52.83 72.05,52.67 71.96,52.58 v68.45,52.58 | R7.2 61.09,59.56 v61.34,59.31
  Top 1.27: 71.75,52.96 72.05,52.67 Q2.D@4 Q2.D@3 75.91,52.67 76.2,52.96 | 76.2,56.26 76.2,57.28 | 76.2,55.63 76.2,56.26 | 76.2,55.12 76.2,55.63 | 76.2,54.48 76.2,55.12 | 76.2,53.98 76.2,54.48 | 76.2,53.98 76.2,52.96 | 75.95,57.53 76.2,57.28 | 75.95,57.53 74.78,57.53 Q2.D@1 | Q2.D@1 Q2.D@2 71.79,57.57 71.5,57.28 | Q1.S@1 Q1.S@2 74.56,58.91 | 74.56,58.91 74.56,57.74 Q2.D@1 | 74.56,58.91 75.95,57.53 | 77.09,57.15 76.33,57.15 76.2,57.28 | 77.72,57.15 77.09,57.15 | J3.P$1 77.72,57.15 | 77.09,57.15 76.2,56.26 | 77.72,57.15 76.2,55.63 | J3.P$1 78.23,57.15 76.2,55.12 | J3.P$1 78.87,57.15 76.2,54.48 | J3.P$1 79.38,57.15 76.2,53.98 | J3.P$1 80.01,56.77 76.2,52.96
  Bottom 0.203: v68.45,52.58 67.69,53.34 v67.06,53.34 61.34,59.05 v61.34,59.31
PHASE-V  (via drill 0.25)
  Top 0.203: U$1.P$41 C2.2 55.31,39.3 56.26,38.35 72.29,38.35 Q4.D@2 | 72.05,34.25 71.21,34.25 70.36,33.4 66.42,33.4 65.28,32.26 63.25,32.26 v62.99,32 | v57.4,26.42 56.52,25.47 R9.2
  Top 1.016: Q3.S@1 Q3.S@2 74.56,40.77 | Q4.D@1 74.56,39.33 74.39,39.15 Q4.D@2
  Top 1.27: 71.75,34.54 72.05,34.25 Q4.D@4 Q4.D@3 74.78,34.29 75.95,34.29 76.45,34.8 | Q4.D@2 75.78,39.15 | 76.33,39.15 75.78,39.15 | 76.33,39.15 79.79,39.15 J4.P$1 | 75.78,39.15 76.45,38.48 76.45,38.1 | 76.45,36.58 76.45,38.1 | 76.45,35.94 76.45,36.58 | 76.45,34.8 76.45,35.94 | J4.P$1 78.61,37.97 76.58,37.97 76.45,38.1 | J4.P$1 77.22,36.58 77.09,36.58 | 77.09,36.58 76.45,36.58 | 77.09,36.58 76.45,35.94 | Q3.S@1 74.56,40.77 | 74.56,40.77 74.56,39.33 | 74.56,40.77 74.71,40.77 76.33,39.15 | J4.P$1 79.5,39.37 78.87,40.01 75.33,40.01 74.56,40.77 | J4.P$1 80.01,38.35 76.45,34.8
  Bottom 0.203: v62.99,32 v57.4,26.42
PHASE-W  (via drill 0.25)
  Top 0.203: C3.2 55.26,36.88 U$1.P$36 52.32,36.88 52.31,36.87 51.73,36.87 v51.31,36.45 | 60.58,20.19 71.7,20.19 71.92,19.98 | v56.64,34.42 57.4,33.66 57.78,33.66 59.05,32.38 59.05,21.72 60.58,20.19 | 60.58,20.19 v59.56,20.19 | v56.26,20.19 53.27,20.19 R14.2
  Top 1.27: Q5.S@1 Q5.S@2 74.56,21.57 | 74.56,21.57 74.56,20.15 Q6.D@1 | Q6.D@1 Q6.D@2 71.92,19.98 71.75,19.81 | Q6.D@1 76.16,19.98 | 76.33,19.81 76.16,19.98 | 76.33,17.78 76.33,19.81 | 76.33,16.64 76.33,17.78 | 76.33,15.37 76.33,16.64 | 76.33,15.37 76.07,15.11 74.78,15.11 Q6.D@3 Q6.D@4 71.92,15.08 71.88,15.11 | 76.16,19.98 78.4,19.98 | 78.4,19.98 77.6,19.18 76.96,19.18 76.33,19.81 | J6.P$1 80.01,20.45 78.23,18.67 | 78.23,18.67 77.22,18.67 76.33,17.78 | 78.23,18.67 78.23,18.54 76.33,16.64 | 74.56,21.57 75.44,20.7 | 75.44,20.7 76.16,19.98 | J6.P$1 78.4,19.98 | 75.44,20.7 79.12,20.7 J6.P$1 | J6.P$1 80.01,19.05 76.33,15.37
  Bottom 0.203: v59.56,20.19 v56.26,20.19 | v51.31,36.45 51.56,36.45 51.82,36.7 54.36,36.7 v56.64,34.42
SHNT-V-HI  (via drill 0.25)
  Top 0.203: R1.SB 62.99,35.43 v63.75,36.2 | v43.05,23.62 R15.1
  Bottom 0.203: v63.75,36.2 64.26,36.2 65.53,34.92 65.53,34.29 64.52,33.27 52.7,33.27 v43.05,23.62
SHNT-V-LO  (via drill 0.25)
  Top 0.203: R1.SA v63.75,42.04 | v44.7,23.62 44.7,24.83 R16.1
  Bottom 0.203: v63.75,42.04 63.75,37.59 66.04,35.31 66.04,34.04 64.77,32.77 52.96,32.77 44.7,24.51 v44.7,23.62
SHNT-W-HI  (via drill 0.25)
  Top 0.203: R17.1 46.86,24.38 47.37,23.88 50.67,23.88 v51.18,24.38 | v62.48,19.25 62.53,19.25 62.99,18.8 62.99,17.59 R10.SB
  Bottom 0.203: v51.18,24.38 51.44,24.38 54.23,21.59 54.23,20.83 55.75,19.3 62.44,19.3 v62.48,19.25
SHNT-W-LO  (via drill 0.25)
  Top 0.203: R10.SA 62.93,22.67 v62.48,22.23 | v51.82,25.02 48.7,25.02 R18.1
  Bottom 0.203: v62.48,22.23 54.61,22.23 v51.82,25.02
SL-V  (via drill 0.25)
  Top 0.203: U$1.P$39 52.19,38.38 v52.07,38.26 | 67.31,35.18 R1.B 65.53,35.43 v64.77,34.67
  Top 1.27: Q4.S@1 Q4.S@2 70.47,36.05 69.6,35.18 67.31,35.18
  Bottom 0.203: v52.07,38.26 54.7,38.26 59.18,33.78 63.88,33.78 v64.77,34.67
SL-W
  Top 0.203: U$1.P$34 54.29,35.88 54.74,35.43 54.74,34.29 55.5,33.53 56.01,33.53 56.11,33.43 56.63,33.43 57.11,32.94 57.48,32.94 58.34,32.08 58.34,16.71 59.56,15.49 63.63,15.49 64.9,16.76 66.55,16.76 67.18,17.4
  Top 1.27: Q6.S@1 Q6.S@2 70.75,16.88 70.23,17.4 67.18,17.4 R10.B
VCC
  pour Top (rank 2): 52.58,66.8 52.58,47.75 51.82,46.99 47.24,46.99 47.24,11.68 101.35,11.68 101.35,66.8

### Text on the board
tPlace: mkbldcdriver v0.1 | U | VCC | GND | USART / GPIO | V | SPI | W | VCC | GND
bPlace: "wow" / - Owen Wilson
